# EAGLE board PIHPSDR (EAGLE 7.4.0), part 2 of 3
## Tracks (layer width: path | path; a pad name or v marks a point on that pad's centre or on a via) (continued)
N$321  (via drill 0.8 pad 1.93)
  other vias: 93.52,31.02
N$322  (via drill 0.8 pad 1.93)
  other vias: 93.52,28.48
N$323  (via drill 0.8 pad 1.93)
  other vias: 93.52,25.94
N$325  (via drill 0.8 pad 1.93)
  other vias: 96.06,119.92
N$326  (via drill 0.8 pad 1.93)
  other vias: 96.06,117.38
N$327  (via drill 0.8 pad 1.93)
  other vias: 96.06,114.84
N$328  (via drill 0.8 pad 1.93)
  other vias: 96.06,112.3
N$329  (via drill 0.8 pad 1.93)
  other vias: 96.06,109.76
N$330  (via drill 0.8 pad 1.93)
  other vias: 96.06,107.22
N$331  (via drill 0.8 pad 1.93)
  other vias: 96.06,104.68
N$332  (via drill 0.8 pad 1.93)
  other vias: 96.06,102.14
N$333  (via drill 0.8 pad 1.93)
  other vias: 96.06,99.6
N$334  (via drill 0.8 pad 1.93)
  other vias: 96.06,97.06
N$335  (via drill 0.8 pad 1.93)
  other vias: 96.06,94.52
N$336  (via drill 0.8 pad 1.93)
  other vias: 96.06,91.98
N$337  (via drill 0.8 pad 1.93)
  other vias: 96.06,89.44
N$338  (via drill 0.8 pad 1.93)
  other vias: 96.06,86.9
N$339  (via drill 0.8 pad 1.93)
  other vias: 96.06,84.36
N$340  (via drill 0.8 pad 1.93)
  other vias: 96.06,81.82
N$341  (via drill 0.8 pad 1.93)
  other vias: 96.06,79.28
N$342  (via drill 0.8 pad 1.93)
  other vias: 96.06,76.74
N$343  (via drill 0.8 pad 1.93)
  other vias: 96.06,74.2
N$344  (via drill 0.8 pad 1.93)
  other vias: 96.06,71.66
N$345  (via drill 0.8 pad 1.93)
  other vias: 96.06,69.12
N$346  (via drill 0.8 pad 1.93)
  other vias: 96.06,66.58
N$347  (via drill 0.8 pad 1.93)
  other vias: 96.06,64.04
N$348  (via drill 0.8 pad 1.93)
  other vias: 96.06,61.5
N$349  (via drill 0.8 pad 1.93)
  other vias: 96.06,58.96
N$350  (via drill 0.8 pad 1.93)
  other vias: 96.06,56.42
N$351  (via drill 0.8 pad 1.93)
  other vias: 96.06,53.88
N$352  (via drill 0.8 pad 1.93)
  other vias: 96.06,51.34
N$353  (via drill 0.8 pad 1.93)
  other vias: 96.06,48.8
N$354  (via drill 0.8 pad 1.93)
  other vias: 96.06,46.26
N$355  (via drill 0.8 pad 1.93)
  other vias: 96.06,43.72
N$356  (via drill 0.8 pad 1.93)
  other vias: 96.06,41.18
N$357  (via drill 0.8 pad 1.93)
  other vias: 96.06,38.64
N$358  (via drill 0.8 pad 1.93)
  other vias: 96.06,36.1
N$359  (via drill 0.8 pad 1.93)
  other vias: 96.06,33.56
N$360  (via drill 0.8 pad 1.93)
  other vias: 96.06,31.02
N$361  (via drill 0.8 pad 1.93)
  other vias: 96.06,28.48
N$362  (via drill 0.8 pad 1.93)
  other vias: 96.06,25.94
N$364  (via drill 0.8 pad 1.93)
  other vias: 98.6,119.92
N$365  (via drill 0.8 pad 1.93)
  other vias: 98.6,117.38
N$366  (via drill 0.8 pad 1.93)
  other vias: 98.6,114.84
N$367  (via drill 0.8 pad 1.93)
  other vias: 98.6,112.3
N$368  (via drill 0.8 pad 1.93)
  other vias: 98.6,109.76
N$369  (via drill 0.8 pad 1.93)
  other vias: 98.6,107.22
N$370  (via drill 0.8 pad 1.93)
  other vias: 98.6,104.68
N$371  (via drill 0.8 pad 1.93)
  other vias: 98.6,102.14
N$372  (via drill 0.8 pad 1.93)
  other vias: 98.6,99.6
N$373  (via drill 0.8 pad 1.93)
  other vias: 98.6,97.06
N$374  (via drill 0.8 pad 1.93)
  other vias: 98.6,94.52
N$375  (via drill 0.8 pad 1.93)
  other vias: 98.6,91.98
N$376  (via drill 0.8 pad 1.93)
  other vias: 98.6,89.44
N$377  (via drill 0.8 pad 1.93)
  other vias: 98.6,86.9
N$378  (via drill 0.8 pad 1.93)
  other vias: 98.6,84.36
N$379  (via drill 0.8 pad 1.93)
  other vias: 98.6,81.82
N$380  (via drill 0.8 pad 1.93)
  other vias: 98.6,79.28
N$381  (via drill 0.8 pad 1.93)
  other vias: 98.6,76.74
N$382  (via drill 0.8 pad 1.93)
  other vias: 98.6,74.2
N$383  (via drill 0.8 pad 1.93)
  other vias: 98.6,71.66
N$384  (via drill 0.8 pad 1.93)
  other vias: 98.6,69.12
N$385  (via drill 0.8 pad 1.93)
  other vias: 98.6,66.58
N$386  (via drill 0.8 pad 1.93)
  other vias: 98.6,64.04
N$387  (via drill 0.8 pad 1.93)
  other vias: 98.6,61.5
N$388  (via drill 0.8 pad 1.93)
  other vias: 98.6,58.96
N$389  (via drill 0.8 pad 1.93)
  other vias: 98.6,56.42
N$390  (via drill 0.8 pad 1.93)
  other vias: 98.6,53.88
N$391  (via drill 0.8 pad 1.93)
  other vias: 98.6,51.34
N$392  (via drill 0.8 pad 1.93)
  other vias: 98.6,48.8
N$393  (via drill 0.8 pad 1.93)
  other vias: 98.6,46.26
N$394  (via drill 0.8 pad 1.93)
  other vias: 98.6,43.72
N$395  (via drill 0.8 pad 1.93)
  other vias: 98.6,41.18
N$396  (via drill 0.8 pad 1.93)
  other vias: 98.6,38.64
N$397  (via drill 0.8 pad 1.93)
  other vias: 98.6,36.1
N$398  (via drill 0.8 pad 1.93)
  other vias: 98.6,33.56
N$399  (via drill 0.8 pad 1.93)
  other vias: 98.6,31.02
N$400  (via drill 0.8 pad 1.93)
  other vias: 98.6,28.48
N$401  (via drill 0.8 pad 1.93)
  other vias: 98.6,25.94
N$403  (via drill 0.8 pad 1.93)
  other vias: 103.68,119.92
N$404  (via drill 0.8 pad 1.93)
  other vias: 103.68,117.38
N$405  (via drill 0.8 pad 1.93)
  other vias: 103.68,114.84
N$406  (via drill 0.8 pad 1.93)
  other vias: 103.68,112.3
N$407  (via drill 0.8 pad 1.93)
  other vias: 103.68,109.76
N$408  (via drill 0.8 pad 1.93)
  other vias: 103.68,107.22
N$409  (via drill 0.8 pad 1.93)
  other vias: 103.68,104.68
N$410  (via drill 0.8 pad 1.93)
  other vias: 103.68,102.14
N$411  (via drill 0.8 pad 1.93)
  other vias: 103.68,99.6
N$412  (via drill 0.8 pad 1.93)
  other vias: 103.68,97.06
N$413  (via drill 0.8 pad 1.93)
  other vias: 103.68,94.52
N$414  (via drill 0.8 pad 1.93)
  other vias: 103.68,91.98
N$415  (via drill 0.8 pad 1.93)
  other vias: 103.68,89.44
N$416  (via drill 0.8 pad 1.93)
  other vias: 103.68,86.9
N$417  (via drill 0.8 pad 1.93)
  other vias: 103.68,84.36
N$418  (via drill 0.8 pad 1.93)
  other vias: 103.68,81.82
N$419  (via drill 0.8 pad 1.93)
  other vias: 103.68,79.28
N$420  (via drill 0.8 pad 1.93)
  other vias: 103.68,76.74
N$421  (via drill 0.8 pad 1.93)
  other vias: 103.68,74.2
N$422  (via drill 0.8 pad 1.93)
  other vias: 103.68,71.66
N$423  (via drill 0.8 pad 1.93)
  other vias: 103.68,69.12
N$424  (via drill 0.8 pad 1.93)
  other vias: 103.68,66.58
N$425  (via drill 0.8 pad 1.93)
  other vias: 103.68,64.04
N$426  (via drill 0.8 pad 1.93)
  other vias: 103.68,61.5
N$427  (via drill 0.8 pad 1.93)
  other vias: 103.68,58.96
N$428  (via drill 0.8 pad 1.93)
  other vias: 103.68,56.42
N$429  (via drill 0.8 pad 1.93)
  other vias: 103.68,53.88
N$430  (via drill 0.8 pad 1.93)
  other vias: 103.68,51.34
N$431  (via drill 0.8 pad 1.93)
  other vias: 103.68,48.8
N$432  (via drill 0.8 pad 1.93)
  other vias: 103.68,46.26
N$433  (via drill 0.8 pad 1.93)
  other vias: 103.68,43.72
N$434  (via drill 0.8 pad 1.93)
  other vias: 103.68,41.18
N$435  (via drill 0.8 pad 1.93)
  other vias: 103.68,38.64
N$436  (via drill 0.8 pad 1.93)
  other vias: 103.68,36.1
N$437  (via drill 0.8 pad 1.93)
  other vias: 103.68,33.56
N$438  (via drill 0.8 pad 1.93)
  other vias: 103.68,31.02
N$439  (via drill 0.8 pad 1.93)
  other vias: 103.68,28.48
N$440  (via drill 0.8 pad 1.93)
  other vias: 103.68,25.94
N$442  (via drill 0.8 pad 1.93)
  other vias: 101.14,119.92
N$443  (via drill 0.8 pad 1.93)
  other vias: 101.14,117.38
N$444  (via drill 0.8 pad 1.93)
  other vias: 101.14,114.84
N$445  (via drill 0.8 pad 1.93)
  other vias: 101.14,112.3
N$446  (via drill 0.8 pad 1.93)
  other vias: 101.14,109.76
N$447  (via drill 0.8 pad 1.93)
  other vias: 101.14,107.22
N$448  (via drill 0.8 pad 1.93)
  other vias: 101.14,104.68
N$449  (via drill 0.8 pad 1.93)
  other vias: 101.14,102.14
N$450  (via drill 0.8 pad 1.93)
  other vias: 101.14,99.6
N$451  (via drill 0.8 pad 1.93)
  other vias: 101.14,97.06
N$452  (via drill 0.8 pad 1.93)
  other vias: 101.14,94.52
N$453  (via drill 0.8 pad 1.93)
  other vias: 101.14,91.98
N$454  (via drill 0.8 pad 1.93)
  other vias: 101.14,89.44
N$455  (via drill 0.8 pad 1.93)
  other vias: 101.14,86.9
N$456  (via drill 0.8 pad 1.93)
  other vias: 101.14,84.36
N$457  (via drill 0.8 pad 1.93)
  other vias: 101.14,81.82
N$458  (via drill 0.8 pad 1.93)
  other vias: 101.14,79.28
N$459  (via drill 0.8 pad 1.93)
  other vias: 101.14,76.74
N$460  (via drill 0.8 pad 1.93)
  other vias: 101.14,74.2
N$461  (via drill 0.8 pad 1.93)
  other vias: 101.14,71.66
N$462  (via drill 0.8 pad 1.93)
  other vias: 101.14,69.12
N$463  (via drill 0.8 pad 1.93)
  other vias: 101.14,66.58
N$464  (via drill 0.8 pad 1.93)
  other vias: 101.14,64.04
N$465  (via drill 0.8 pad 1.93)
  other vias: 101.14,61.5
N$466  (via drill 0.8 pad 1.93)
  other vias: 101.14,58.96
N$467  (via drill 0.8 pad 1.93)
  other vias: 101.14,56.42
N$468  (via drill 0.8 pad 1.93)
  other vias: 101.14,53.88
N$469  (via drill 0.8 pad 1.93)
  other vias: 101.14,51.34
N$470  (via drill 0.8 pad 1.93)
  other vias: 101.14,48.8
N$471  (via drill 0.8 pad 1.93)
  other vias: 101.14,46.26
N$472  (via drill 0.8 pad 1.93)
  other vias: 101.14,43.72
N$473  (via drill 0.8 pad 1.93)
  other vias: 101.14,41.18
N$474  (via drill 0.8 pad 1.93)
  other vias: 101.14,38.64
N$475  (via drill 0.8 pad 1.93)
  other vias: 101.14,36.1
N$476  (via drill 0.8 pad 1.93)
  other vias: 101.14,33.56
N$477  (via drill 0.8 pad 1.93)
  other vias: 101.14,31.02
N$478  (via drill 0.8 pad 1.93)
  other vias: 101.14,28.48
N$479  (via drill 0.8 pad 1.93)
  other vias: 101.14,25.94
N$481  (via drill 0.8 pad 1.93)
  other vias: 106.22,119.92
N$482  (via drill 0.8 pad 1.93)
  other vias: 106.22,117.38
N$483  (via drill 0.8 pad 1.93)
  other vias: 106.22,114.84
N$484  (via drill 0.8 pad 1.93)
  other vias: 106.22,112.3
N$485  (via drill 0.8 pad 1.93)
  other vias: 106.22,109.76
N$486  (via drill 0.8 pad 1.93)
  other vias: 106.22,107.22
N$487  (via drill 0.8 pad 1.93)
  other vias: 106.22,104.68
N$488  (via drill 0.8 pad 1.93)
  other vias: 106.22,102.14
N$489  (via drill 0.8 pad 1.93)
  other vias: 106.22,99.6
N$490  (via drill 0.8 pad 1.93)
  other vias: 106.22,97.06
N$491  (via drill 0.8 pad 1.93)
  other vias: 106.22,94.52
N$492  (via drill 0.8 pad 1.93)
  other vias: 106.22,91.98
N$493  (via drill 0.8 pad 1.93)
  other vias: 106.22,89.44
N$494  (via drill 0.8 pad 1.93)
  other vias: 106.22,86.9
N$495  (via drill 0.8 pad 1.93)
  other vias: 106.22,84.36
N$496  (via drill 0.8 pad 1.93)
  other vias: 106.22,81.82
N$497  (via drill 0.8 pad 1.93)
  other vias: 106.22,79.28
N$498  (via drill 0.8 pad 1.93)
  other vias: 106.22,76.74
N$499  (via drill 0.8 pad 1.93)
  other vias: 106.22,74.2
N$500  (via drill 0.8 pad 1.93)
  other vias: 106.22,71.66
N$501  (via drill 0.8 pad 1.93)
  other vias: 106.22,69.12
N$502  (via drill 0.8 pad 1.93)
  other vias: 106.22,66.58
N$503  (via drill 0.8 pad 1.93)
  other vias: 106.22,64.04
N$504  (via drill 0.8 pad 1.93)
  other vias: 106.22,61.5
N$505  (via drill 0.8 pad 1.93)
  other vias: 106.22,58.96
N$506  (via drill 0.8 pad 1.93)
  other vias: 106.22,56.42
N$507  (via drill 0.8 pad 1.93)
  other vias: 106.22,53.88
N$508  (via drill 0.8 pad 1.93)
  other vias: 106.22,51.34
N$509  (via drill 0.8 pad 1.93)
  other vias: 106.22,48.8
N$510  (via drill 0.8 pad 1.93)
  other vias: 106.22,46.26
N$511  (via drill 0.8 pad 1.93)
  other vias: 106.22,43.72
N$512  (via drill 0.8 pad 1.93)
  other vias: 106.22,41.18
N$513  (via drill 0.8 pad 1.93)
  other vias: 106.22,38.64
N$514  (via drill 0.8 pad 1.93)
  other vias: 106.22,36.1
N$515  (via drill 0.8 pad 1.93)
  other vias: 106.22,33.56
N$516  (via drill 0.8 pad 1.93)
  other vias: 106.22,31.02
N$517  (via drill 0.8 pad 1.93)
  other vias: 106.22,28.48
N$518  (via drill 0.8 pad 1.93)
  other vias: 106.22,25.94
N$520  (via drill 0.8 pad 1.93)
  other vias: 108.76,119.92
N$521  (via drill 0.8 pad 1.93)
  other vias: 108.76,117.38
N$522  (via drill 0.8 pad 1.93)
  other vias: 108.76,114.84
N$523  (via drill 0.8 pad 1.93)
  other vias: 108.76,112.3
N$524  (via drill 0.8 pad 1.93)
  other vias: 108.76,109.76
N$525  (via drill 0.8 pad 1.93)
  other vias: 108.76,107.22
N$526  (via drill 0.8 pad 1.93)
  other vias: 108.76,104.68
N$527  (via drill 0.8 pad 1.93)
  other vias: 108.76,102.14
N$528  (via drill 0.8 pad 1.93)
  other vias: 108.76,99.6
N$529  (via drill 0.8 pad 1.93)
  other vias: 108.76,97.06
N$530  (via drill 0.8 pad 1.93)
  other vias: 108.76,94.52
N$531  (via drill 0.8 pad 1.93)
  other vias: 108.76,91.98
N$532  (via drill 0.8 pad 1.93)
  other vias: 108.76,89.44
N$533  (via drill 0.8 pad 1.93)
  other vias: 108.76,86.9
N$534  (via drill 0.8 pad 1.93)
  other vias: 108.76,84.36
N$535  (via drill 0.8 pad 1.93)
  other vias: 108.76,81.82
N$536  (via drill 0.8 pad 1.93)
  other vias: 108.76,79.28
N$537  (via drill 0.8 pad 1.93)
  other vias: 108.76,76.74
N$538  (via drill 0.8 pad 1.93)
  other vias: 108.76,74.2
N$539  (via drill 0.8 pad 1.93)
  other vias: 108.76,71.66
N$540  (via drill 0.8 pad 1.93)
  other vias: 108.76,69.12
N$541  (via drill 0.8 pad 1.93)
  other vias: 108.76,66.58
N$542  (via drill 0.8 pad 1.93)
  other vias: 108.76,64.04
N$543  (via drill 0.8 pad 1.93)
  other vias: 108.76,61.5
N$544  (via drill 0.8 pad 1.93)
  other vias: 108.76,58.96
N$545  (via drill 0.8 pad 1.93)
  other vias: 108.76,56.42
N$546  (via drill 0.8 pad 1.93)
  other vias: 108.76,53.88
N$547  (via drill 0.8 pad 1.93)
  other vias: 108.76,51.34
N$548  (via drill 0.8 pad 1.93)
  other vias: 108.76,48.8
N$549  (via drill 0.8 pad 1.93)
  other vias: 108.76,46.26
N$550  (via drill 0.8 pad 1.93)
  other vias: 108.76,43.72
N$551  (via drill 0.8 pad 1.93)
  other vias: 108.76,41.18
N$552  (via drill 0.8 pad 1.93)
  other vias: 108.76,38.64
N$553  (via drill 0.8 pad 1.93)
  other vias: 108.76,36.1
N$554  (via drill 0.8 pad 1.93)
  other vias: 108.76,33.56
N$555  (via drill 0.8 pad 1.93)
  other vias: 108.76,31.02
N$556  (via drill 0.8 pad 1.93)
  other vias: 108.76,28.48
N$557  (via drill 0.8 pad 1.93)
  other vias: 108.76,25.94
N$559  (via drill 0.8 pad 1.93)
  other vias: 111.3,119.92
N$560  (via drill 0.8 pad 1.93)
  other vias: 111.3,117.38
N$561  (via drill 0.8 pad 1.93)
  other vias: 111.3,114.84
N$562  (via drill 0.8 pad 1.93)
  other vias: 111.3,112.3
N$563  (via drill 0.8 pad 1.93)
  other vias: 111.3,109.76
N$564  (via drill 0.8 pad 1.93)
  other vias: 111.3,107.22
N$565  (via drill 0.8 pad 1.93)
  other vias: 111.3,104.68
N$566  (via drill 0.8 pad 1.93)
  other vias: 111.3,102.14
N$567  (via drill 0.8 pad 1.93)
  other vias: 111.3,99.6
N$568  (via drill 0.8 pad 1.93)
  other vias: 111.3,97.06
N$569  (via drill 0.8 pad 1.93)
  other vias: 111.3,94.52
N$570  (via drill 0.8 pad 1.93)
  other vias: 111.3,91.98
N$571  (via drill 0.8 pad 1.93)
  other vias: 111.3,89.44
N$572  (via drill 0.8 pad 1.93)
  other vias: 111.3,86.9
N$573  (via drill 0.8 pad 1.93)
  other vias: 111.3,84.36
N$574  (via drill 0.8 pad 1.93)
  other vias: 111.3,81.82
N$575  (via drill 0.8 pad 1.93)
  other vias: 111.3,79.28
N$576  (via drill 0.8 pad 1.93)
  other vias: 111.3,76.74
N$577  (via drill 0.8 pad 1.93)
  other vias: 111.3,74.2
N$578  (via drill 0.8 pad 1.93)
  other vias: 111.3,71.66
N$579  (via drill 0.8 pad 1.93)
  other vias: 111.3,69.12
N$580  (via drill 0.8 pad 1.93)
  other vias: 111.3,66.58
N$581  (via drill 0.8 pad 1.93)
  other vias: 111.3,64.04
N$582  (via drill 0.8 pad 1.93)
  other vias: 111.3,61.5
N$583  (via drill 0.8 pad 1.93)
  other vias: 111.3,58.96
N$584  (via drill 0.8 pad 1.93)
  other vias: 111.3,56.42
N$585  (via drill 0.8 pad 1.93)
  other vias: 111.3,53.88
N$586  (via drill 0.8 pad 1.93)
  other vias: 111.3,51.34
N$587  (via drill 0.8 pad 1.93)
  other vias: 111.3,48.8
N$588  (via drill 0.8 pad 1.93)
  other vias: 111.3,46.26
N$589  (via drill 0.8 pad 1.93)
  other vias: 111.3,43.72
N$590  (via drill 0.8 pad 1.93)
  other vias: 111.3,41.18
N$591  (via drill 0.8 pad 1.93)
  other vias: 111.3,38.64
N$592  (via drill 0.8 pad 1.93)
  other vias: 111.3,36.1
N$593  (via drill 0.8 pad 1.93)
  other vias: 111.3,33.56
N$594  (via drill 0.8 pad 1.93)
  other vias: 111.3,31.02
N$595  (via drill 0.8 pad 1.93)
  other vias: 111.3,28.48
N$596  (via drill 0.8 pad 1.93)
  other vias: 111.3,25.94
N$598  (via drill 0.8 pad 1.93)
  other vias: 113.84,119.92
N$599  (via drill 0.8 pad 1.93)
  other vias: 113.84,117.38
N$600  (via drill 0.8 pad 1.93)
  other vias: 113.84,114.84
N$601  (via drill 0.8 pad 1.93)
  other vias: 113.84,112.3
N$602  (via drill 0.8 pad 1.93)
  other vias: 113.84,109.76
N$603  (via drill 0.8 pad 1.93)
  other vias: 113.84,107.22
N$604  (via drill 0.8 pad 1.93)
  other vias: 113.84,104.68
N$605  (via drill 0.8 pad 1.93)
  other vias: 113.84,102.14
N$606  (via drill 0.8 pad 1.93)
  other vias: 113.84,99.6
N$607  (via drill 0.8 pad 1.93)
  other vias: 113.84,97.06
N$608  (via drill 0.8 pad 1.93)
  other vias: 113.84,94.52
N$609  (via drill 0.8 pad 1.93)
  other vias: 113.84,91.98
N$610  (via drill 0.8 pad 1.93)
  other vias: 113.84,89.44
N$611  (via drill 0.8 pad 1.93)
  other vias: 113.84,86.9
N$612  (via drill 0.8 pad 1.93)
  other vias: 113.84,84.36
N$613  (via drill 0.8 pad 1.93)
  other vias: 113.84,81.82
N$614  (via drill 0.8 pad 1.93)
  other vias: 113.84,79.28
N$615  (via drill 0.8 pad 1.93)
  other vias: 113.84,76.74
N$616  (via drill 0.8 pad 1.93)
  other vias: 113.84,74.2
N$617  (via drill 0.8 pad 1.93)
  other vias: 113.84,71.66
N$618  (via drill 0.8 pad 1.93)
  other vias: 113.84,69.12
N$619  (via drill 0.8 pad 1.93)
  other vias: 113.84,66.58
N$620  (via drill 0.8 pad 1.93)
  other vias: 113.84,64.04
N$621  (via drill 0.8 pad 1.93)
  other vias: 113.84,61.5
N$622  (via drill 0.8 pad 1.93)
  other vias: 113.84,58.96
N$623  (via drill 0.8 pad 1.93)
  other vias: 113.84,56.42
N$624  (via drill 0.8 pad 1.93)
  other vias: 113.84,53.88
N$625  (via drill 0.8 pad 1.93)
  other vias: 113.84,51.34
N$626  (via drill 0.8 pad 1.93)
  other vias: 113.84,48.8
N$627  (via drill 0.8 pad 1.93)
  other vias: 113.84,46.26
N$628  (via drill 0.8 pad 1.93)
  other vias: 113.84,43.72
N$629  (via drill 0.8 pad 1.93)
  other vias: 113.84,41.18
N$630  (via drill 0.8 pad 1.93)
  other vias: 113.84,38.64
N$631  (via drill 0.8 pad 1.93)
  other vias: 113.84,36.1
N$632  (via drill 0.8 pad 1.93)
  other vias: 113.84,33.56
N$633  (via drill 0.8 pad 1.93)
  other vias: 113.84,31.02
N$634  (via drill 0.8 pad 1.93)
  other vias: 113.84,28.48
N$635  (via drill 0.8 pad 1.93)
  other vias: 113.84,25.94
N$637  (via drill 0.8 pad 1.93)
  other vias: 116.38,119.92
N$638  (via drill 0.8 pad 1.93)
  other vias: 116.38,117.38
N$639  (via drill 0.8 pad 1.93)
  other vias: 116.38,114.84
N$640  (via drill 0.8 pad 1.93)
  other vias: 116.38,112.3
N$641  (via drill 0.8 pad 1.93)
  other vias: 116.38,109.76
N$642  (via drill 0.8 pad 1.93)
  other vias: 116.38,107.22
N$643  (via drill 0.8 pad 1.93)
  other vias: 116.38,104.68
N$644  (via drill 0.8 pad 1.93)
  other vias: 116.38,102.14
N$645  (via drill 0.8 pad 1.93)
  other vias: 116.38,99.6
N$646  (via drill 0.8 pad 1.93)
  other vias: 116.38,97.06
N$647  (via drill 0.8 pad 1.93)
  other vias: 116.38,94.52
N$648  (via drill 0.8 pad 1.93)
  other vias: 116.38,91.98
N$649  (via drill 0.8 pad 1.93)
  other vias: 116.38,89.44
N$650  (via drill 0.8 pad 1.93)
  other vias: 116.38,86.9
N$651  (via drill 0.8 pad 1.93)
  other vias: 116.38,84.36
N$652  (via drill 0.8 pad 1.93)
  other vias: 116.38,81.82
N$653  (via drill 0.8 pad 1.93)
  other vias: 116.38,79.28
N$654  (via drill 0.8 pad 1.93)
  other vias: 116.38,76.74
N$655  (via drill 0.8 pad 1.93)
  other vias: 116.38,74.2
N$656  (via drill 0.8 pad 1.93)
  other vias: 116.38,71.66
N$657  (via drill 0.8 pad 1.93)
  other vias: 116.38,69.12
N$658  (via drill 0.8 pad 1.93)
  other vias: 116.38,66.58
N$659  (via drill 0.8 pad 1.93)
  other vias: 116.38,64.04
N$660  (via drill 0.8 pad 1.93)
  other vias: 116.38,61.5
N$661  (via drill 0.8 pad 1.93)
  other vias: 116.38,58.96
N$662  (via drill 0.8 pad 1.93)
  other vias: 116.38,56.42
N$663  (via drill 0.8 pad 1.93)
  other vias: 116.38,53.88
N$664  (via drill 0.8 pad 1.93)
  other vias: 116.38,51.34
N$665  (via drill 0.8 pad 1.93)
  other vias: 116.38,48.8
N$666  (via drill 0.8 pad 1.93)
  other vias: 116.38,46.26
N$667  (via drill 0.8 pad 1.93)
  other vias: 116.38,43.72
N$668  (via drill 0.8 pad 1.93)
  other vias: 116.38,41.18
N$669  (via drill 0.8 pad 1.93)
  other vias: 116.38,38.64
N$670  (via drill 0.8 pad 1.93)
  other vias: 116.38,36.1
N$671  (via drill 0.8 pad 1.93)
  other vias: 116.38,33.56
N$672  (via drill 0.8 pad 1.93)
  other vias: 116.38,31.02
N$673  (via drill 0.8 pad 1.93)
  other vias: 116.38,28.48
N$674  (via drill 0.8 pad 1.93)
  other vias: 116.38,25.94
N$676  (via drill 0.8 pad 1.93)
  other vias: 118.92,119.92
N$677  (via drill 0.8 pad 1.93)
  other vias: 118.92,117.38
N$678  (via drill 0.8 pad 1.93)
  other vias: 118.92,114.84
N$679  (via drill 0.8 pad 1.93)
  other vias: 118.92,112.3
N$680  (via drill 0.8 pad 1.93)
  other vias: 118.92,109.76
N$681  (via drill 0.8 pad 1.93)
  other vias: 118.92,107.22
N$682  (via drill 0.8 pad 1.93)
  other vias: 118.92,104.68
N$683  (via drill 0.8 pad 1.93)
  other vias: 118.92,102.14
N$684  (via drill 0.8 pad 1.93)
  other vias: 118.92,99.6
N$685  (via drill 0.8 pad 1.93)
  other vias: 118.92,97.06
N$686  (via drill 0.8 pad 1.93)
  other vias: 118.92,94.52
N$687  (via drill 0.8 pad 1.93)
  other vias: 118.92,91.98
N$688  (via drill 0.8 pad 1.93)
  other vias: 118.92,89.44
N$689  (via drill 0.8 pad 1.93)
  other vias: 118.92,86.9
N$690  (via drill 0.8 pad 1.93)
  other vias: 118.92,84.36
N$691  (via drill 0.8 pad 1.93)
  other vias: 118.92,81.82
N$692  (via drill 0.8 pad 1.93)
  other vias: 118.92,79.28
N$693  (via drill 0.8 pad 1.93)
  other vias: 118.92,76.74
N$694  (via drill 0.8 pad 1.93)
  other vias: 118.92,74.2
N$695  (via drill 0.8 pad 1.93)
  other vias: 118.92,71.66
N$696  (via drill 0.8 pad 1.93)
  other vias: 118.92,69.12
N$697  (via drill 0.8 pad 1.93)
  other vias: 118.92,66.58
N$698  (via drill 0.8 pad 1.93)
  other vias: 118.92,64.04
N$699  (via drill 0.8 pad 1.93)
  other vias: 118.92,61.5
N$700  (via drill 0.8 pad 1.93)
  other vias: 118.92,58.96
N$701  (via drill 0.8 pad 1.93)
  other vias: 118.92,56.42
N$702  (via drill 0.8 pad 1.93)
  other vias: 118.92,53.88
N$703  (via drill 0.8 pad 1.93)
  other vias: 118.92,51.34
N$704  (via drill 0.8 pad 1.93)
  other vias: 118.92,48.8
N$705  (via drill 0.8 pad 1.93)
  other vias: 118.92,46.26
N$706  (via drill 0.8 pad 1.93)
  other vias: 118.92,43.72
N$707  (via drill 0.8 pad 1.93)
  other vias: 118.92,41.18
N$708  (via drill 0.8 pad 1.93)
  other vias: 118.92,38.64
N$709  (via drill 0.8 pad 1.93)
  other vias: 118.92,36.1
N$710  (via drill 0.8 pad 1.93)
  other vias: 118.92,33.56
N$711  (via drill 0.8 pad 1.93)
  other vias: 118.92,31.02
N$712  (via drill 0.8 pad 1.93)
  other vias: 118.92,28.48
N$713  (via drill 0.8 pad 1.93)
  other vias: 118.92,25.94
N$715  (via drill 0.8 pad 1.93)
  other vias: 121.46,119.92
N$716  (via drill 0.8 pad 1.93)
  other vias: 121.46,117.38
N$717  (via drill 0.8 pad 1.93)
  other vias: 121.46,114.84
N$718  (via drill 0.8 pad 1.93)
  other vias: 121.46,112.3
N$719  (via drill 0.8 pad 1.93)
  other vias: 121.46,109.76
N$720  (via drill 0.8 pad 1.93)
  other vias: 121.46,107.22
N$721  (via drill 0.8 pad 1.93)
  other vias: 121.46,104.68
N$722  (via drill 0.8 pad 1.93)
  other vias: 121.46,102.14
N$723  (via drill 0.8 pad 1.93)
  other vias: 121.46,99.6
N$724  (via drill 0.8 pad 1.93)
  other vias: 121.46,97.06
N$725  (via drill 0.8 pad 1.93)
  other vias: 121.46,94.52
N$726  (via drill 0.8 pad 1.93)
  other vias: 121.46,91.98
N$727  (via drill 0.8 pad 1.93)
  other vias: 121.46,89.44
N$728  (via drill 0.8 pad 1.93)
  other vias: 121.46,86.9
N$729  (via drill 0.8 pad 1.93)
  other vias: 121.46,84.36
N$730  (via drill 0.8 pad 1.93)
  other vias: 121.46,81.82
N$731  (via drill 0.8 pad 1.93)
  other vias: 121.46,79.28
N$732  (via drill 0.8 pad 1.93)
  other vias: 121.46,76.74
N$733  (via drill 0.8 pad 1.93)
  other vias: 121.46,74.2
N$734  (via drill 0.8 pad 1.93)
  other vias: 121.46,71.66
N$735  (via drill 0.8 pad 1.93)
  other vias: 121.46,69.12
N$736  (via drill 0.8 pad 1.93)
  other vias: 121.46,66.58
N$737  (via drill 0.8 pad 1.93)
  other vias: 121.46,64.04
N$738  (via drill 0.8 pad 1.93)
  other vias: 121.46,61.5
N$739  (via drill 0.8 pad 1.93)
  other vias: 121.46,58.96
N$740  (via drill 0.8 pad 1.93)
  other vias: 121.46,56.42
N$741  (via drill 0.8 pad 1.93)
  other vias: 121.46,53.88
N$742  (via drill 0.8 pad 1.93)
  other vias: 121.46,51.34
N$743  (via drill 0.8 pad 1.93)
  other vias: 121.46,48.8
N$744  (via drill 0.8 pad 1.93)
  other vias: 121.46,46.26
N$745  (via drill 0.8 pad 1.93)
  other vias: 121.46,43.72
N$746  (via drill 0.8 pad 1.93)
  other vias: 121.46,41.18
N$747  (via drill 0.8 pad 1.93)
  other vias: 121.46,38.64
N$748  (via drill 0.8 pad 1.93)
  other vias: 121.46,36.1
N$749  (via drill 0.8 pad 1.93)
  other vias: 121.46,33.56
N$750  (via drill 0.8 pad 1.93)
  other vias: 121.46,31.02
N$751  (via drill 0.8 pad 1.93)
  other vias: 121.46,28.48
N$752  (via drill 0.8 pad 1.93)
  other vias: 121.46,25.94
N$754  (via drill 0.8 pad 1.93)
  other vias: 126.54,119.92
N$755  (via drill 0.8 pad 1.93)
  other vias: 126.54,117.38
N$756  (via drill 0.8 pad 1.93)
  other vias: 126.54,114.84
N$757  (via drill 0.8 pad 1.93)
  other vias: 126.54,112.3
N$758  (via drill 0.8 pad 1.93)
  other vias: 126.54,109.76
N$759  (via drill 0.8 pad 1.93)
  other vias: 126.54,107.22
N$760  (via drill 0.8 pad 1.93)
  other vias: 126.54,104.68
N$761  (via drill 0.8 pad 1.93)
  other vias: 126.54,102.14
N$762  (via drill 0.8 pad 1.93)
  other vias: 126.54,99.6
N$763  (via drill 0.8 pad 1.93)
  other vias: 126.54,97.06
N$764  (via drill 0.8 pad 1.93)
  other vias: 126.54,94.52
N$765  (via drill 0.8 pad 1.93)
  other vias: 126.54,91.98
N$766  (via drill 0.8 pad 1.93)
  other vias: 126.54,89.44
N$767  (via drill 0.8 pad 1.93)
  other vias: 126.54,86.9
N$768  (via drill 0.8 pad 1.93)
  other vias: 126.54,84.36
N$769  (via drill 0.8 pad 1.93)
  other vias: 126.54,81.82
N$770  (via drill 0.8 pad 1.93)
  other vias: 126.54,79.28
N$771  (via drill 0.8 pad 1.93)
  other vias: 126.54,76.74
N$772  (via drill 0.8 pad 1.93)
  other vias: 126.54,74.2
N$773  (via drill 0.8 pad 1.93)
  other vias: 126.54,71.66
N$774  (via drill 0.8 pad 1.93)
  other vias: 126.54,69.12
N$775  (via drill 0.8 pad 1.93)
  other vias: 126.54,66.58
N$776  (via drill 0.8 pad 1.93)
  other vias: 126.54,64.04
N$777  (via drill 0.8 pad 1.93)
  other vias: 126.54,61.5
N$778  (via drill 0.8 pad 1.93)
  other vias: 126.54,58.96
N$779  (via drill 0.8 pad 1.93)
  other vias: 126.54,56.42
N$780  (via drill 0.8 pad 1.93)
  other vias: 126.54,53.88
N$781  (via drill 0.8 pad 1.93)
  other vias: 126.54,51.34
N$782  (via drill 0.8 pad 1.93)
  other vias: 126.54,48.8
N$783  (via drill 0.8 pad 1.93)
  other vias: 126.54,46.26
N$784  (via drill 0.8 pad 1.93)
  other vias: 126.54,43.72
N$785  (via drill 0.8 pad 1.93)
  other vias: 126.54,41.18
N$786  (via drill 0.8 pad 1.93)
  other vias: 126.54,38.64
N$787  (via drill 0.8 pad 1.93)
  other vias: 126.54,36.1
N$788  (via drill 0.8 pad 1.93)
  other vias: 126.54,33.56
N$789  (via drill 0.8 pad 1.93)
  other vias: 126.54,31.02
N$790  (via drill 0.8 pad 1.93)
  other vias: 126.54,28.48
N$791  (via drill 0.8 pad 1.93)
  other vias: 126.54,25.94
N$793  (via drill 0.8 pad 1.93)
  other vias: 124,119.92
N$794  (via drill 0.8 pad 1.93)
  other vias: 124,117.38
N$795  (via drill 0.8 pad 1.93)
  other vias: 124,114.84
N$796  (via drill 0.8 pad 1.93)
  other vias: 124,112.3
N$797  (via drill 0.8 pad 1.93)
  other vias: 124,109.76
N$798  (via drill 0.8 pad 1.93)
  other vias: 124,107.22
N$799  (via drill 0.8 pad 1.93)
  other vias: 124,104.68
N$800  (via drill 0.8 pad 1.93)
  other vias: 124,102.14
N$801  (via drill 0.8 pad 1.93)
  other vias: 124,99.6
N$802  (via drill 0.8 pad 1.93)
  other vias: 124,97.06
N$803  (via drill 0.8 pad 1.93)
  other vias: 124,94.52
N$804  (via drill 0.8 pad 1.93)
  other vias: 124,91.98
N$805  (via drill 0.8 pad 1.93)
  other vias: 124,89.44
N$806  (via drill 0.8 pad 1.93)
  other vias: 124,86.9
N$807  (via drill 0.8 pad 1.93)
  other vias: 124,84.36
N$808  (via drill 0.8 pad 1.93)
  other vias: 124,81.82
N$809  (via drill 0.8 pad 1.93)
  other vias: 124,79.28
N$810  (via drill 0.8 pad 1.93)
  other vias: 124,76.74
N$811  (via drill 0.8 pad 1.93)
  other vias: 124,74.2
N$812  (via drill 0.8 pad 1.93)
  other vias: 124,71.66
N$813  (via drill 0.8 pad 1.93)
  other vias: 124,69.12
N$814  (via drill 0.8 pad 1.93)
  other vias: 124,66.58
N$815  (via drill 0.8 pad 1.93)
  other vias: 124,64.04
N$816  (via drill 0.8 pad 1.93)
  other vias: 124,61.5
N$817  (via drill 0.8 pad 1.93)
  other vias: 124,58.96
N$818  (via drill 0.8 pad 1.93)
  other vias: 124,56.42
N$819  (via drill 0.8 pad 1.93)
  other vias: 124,53.88
N$820  (via drill 0.8 pad 1.93)
  other vias: 124,51.34
N$821  (via drill 0.8 pad 1.93)
  other vias: 124,48.8
N$822  (via drill 0.8 pad 1.93)
  other vias: 124,46.26
N$823  (via drill 0.8 pad 1.93)
  other vias: 124,43.72
N$824  (via drill 0.8 pad 1.93)
  other vias: 124,41.18
N$825  (via drill 0.8 pad 1.93)
  other vias: 124,38.64
N$826  (via drill 0.8 pad 1.93)
  other vias: 124,36.1
N$827  (via drill 0.8 pad 1.93)
  other vias: 124,33.56
N$828  (via drill 0.8 pad 1.93)
  other vias: 124,31.02
N$829  (via drill 0.8 pad 1.93)
  other vias: 124,28.48
N$830  (via drill 0.8 pad 1.93)
  other vias: 124,25.94
N$832  (via drill 0.8 pad 1.93)
  other vias: 129.08,119.92
N$833  (via drill 0.8 pad 1.93)
  other vias: 129.08,117.38
N$834  (via drill 0.8 pad 1.93)
  other vias: 129.08,114.84
N$835  (via drill 0.8 pad 1.93)
  other vias: 129.08,112.3
N$836  (via drill 0.8 pad 1.93)
  other vias: 129.08,109.76
N$837  (via drill 0.8 pad 1.93)
  other vias: 129.08,107.22
N$838  (via drill 0.8 pad 1.93)
  other vias: 129.08,104.68
N$839  (via drill 0.8 pad 1.93)
  other vias: 129.08,102.14
N$840  (via drill 0.8 pad 1.93)
  other vias: 129.08,99.6
N$841  (via drill 0.8 pad 1.93)
  other vias: 129.08,97.06
N$842  (via drill 0.8 pad 1.93)
  other vias: 129.08,94.52
N$843  (via drill 0.8 pad 1.93)
  other vias: 129.08,91.98
N$844  (via drill 0.8 pad 1.93)
  other vias: 129.08,89.44
N$845  (via drill 0.8 pad 1.93)
  other vias: 129.08,86.9
N$846  (via drill 0.8 pad 1.93)
  other vias: 129.08,84.36
N$847  (via drill 0.8 pad 1.93)
  other vias: 129.08,81.82
N$848  (via drill 0.8 pad 1.93)
  other vias: 129.08,79.28
N$849  (via drill 0.8 pad 1.93)
  other vias: 129.08,76.74
N$850  (via drill 0.8 pad 1.93)
  other vias: 129.08,74.2
N$851  (via drill 0.8 pad 1.93)
  other vias: 129.08,71.66
N$852  (via drill 0.8 pad 1.93)
  other vias: 129.08,69.12
N$853  (via drill 0.8 pad 1.93)
  other vias: 129.08,66.58
N$854  (via drill 0.8 pad 1.93)
  other vias: 129.08,64.04
N$855  (via drill 0.8 pad 1.93)
  other vias: 129.08,61.5
N$856  (via drill 0.8 pad 1.93)
  other vias: 129.08,58.96
N$857  (via drill 0.8 pad 1.93)
  other vias: 129.08,56.42
N$858  (via drill 0.8 pad 1.93)
  other vias: 129.08,53.88
N$859  (via drill 0.8 pad 1.93)
  other vias: 129.08,51.34
N$860  (via drill 0.8 pad 1.93)
  other vias: 129.08,48.8
N$861  (via drill 0.8 pad 1.93)
  other vias: 129.08,46.26
N$862  (via drill 0.8 pad 1.93)
  other vias: 129.08,43.72
N$863  (via drill 0.8 pad 1.93)
  other vias: 129.08,41.18
N$864  (via drill 0.8 pad 1.93)
  other vias: 129.08,38.64
N$865  (via drill 0.8 pad 1.93)
  other vias: 129.08,36.1
N$866  (via drill 0.8 pad 1.93)
  other vias: 129.08,33.56
N$867  (via drill 0.8 pad 1.93)
  other vias: 129.08,31.02
N$868  (via drill 0.8 pad 1.93)
  other vias: 129.08,28.48
N$869  (via drill 0.8 pad 1.93)
  other vias: 129.08,25.94
N$871  (via drill 0.8 pad 1.93)
  other vias: 131.62,119.92
N$872  (via drill 0.8 pad 1.93)
  other vias: 131.62,117.38
N$873  (via drill 0.8 pad 1.93)
  other vias: 131.62,114.84
N$874  (via drill 0.8 pad 1.93)
  other vias: 131.62,112.3
N$875  (via drill 0.8 pad 1.93)
  other vias: 131.62,109.76
N$876  (via drill 0.8 pad 1.93)
  other vias: 131.62,107.22
N$877  (via drill 0.8 pad 1.93)
  other vias: 131.62,104.68
N$878  (via drill 0.8 pad 1.93)
  other vias: 131.62,102.14
N$879  (via drill 0.8 pad 1.93)
  other vias: 131.62,99.6
N$880  (via drill 0.8 pad 1.93)
  other vias: 131.62,97.06
N$881  (via drill 0.8 pad 1.93)
  other vias: 131.62,94.52
N$882  (via drill 0.8 pad 1.93)
  other vias: 131.62,91.98
N$883  (via drill 0.8 pad 1.93)
  other vias: 131.62,89.44
N$884  (via drill 0.8 pad 1.93)
  other vias: 131.62,86.9
N$885  (via drill 0.8 pad 1.93)
  other vias: 131.62,84.36
N$886  (via drill 0.8 pad 1.93)
  other vias: 131.62,81.82
N$887  (via drill 0.8 pad 1.93)
  other vias: 131.62,79.28
N$888  (via drill 0.8 pad 1.93)
  other vias: 131.62,76.74
N$889  (via drill 0.8 pad 1.93)
  other vias: 131.62,74.2
N$890  (via drill 0.8 pad 1.93)
  other vias: 131.62,71.66
N$891  (via drill 0.8 pad 1.93)
  other vias: 131.62,69.12
N$892  (via drill 0.8 pad 1.93)
  other vias: 131.62,66.58
N$893  (via drill 0.8 pad 1.93)
  other vias: 131.62,64.04
N$894  (via drill 0.8 pad 1.93)
  other vias: 131.62,61.5
N$895  (via drill 0.8 pad 1.93)
  other vias: 131.62,58.96
N$896  (via drill 0.8 pad 1.93)
  other vias: 131.62,56.42
N$897  (via drill 0.8 pad 1.93)
  other vias: 131.62,53.88
N$898  (via drill 0.8 pad 1.93)
  other vias: 131.62,51.34
N$899  (via drill 0.8 pad 1.93)
  other vias: 131.62,48.8
N$900  (via drill 0.8 pad 1.93)
  other vias: 131.62,46.26
N$901  (via drill 0.8 pad 1.93)
  other vias: 131.62,43.72
N$902  (via drill 0.8 pad 1.93)
  other vias: 131.62,41.18
N$903  (via drill 0.8 pad 1.93)
  other vias: 131.62,38.64
N$904  (via drill 0.8 pad 1.93)
  other vias: 131.62,36.1
N$905  (via drill 0.8 pad 1.93)
  other vias: 131.62,33.56
N$906  (via drill 0.8 pad 1.93)
  other vias: 131.62,31.02
N$907  (via drill 0.8 pad 1.93)
  other vias: 131.62,28.48
N$908  (via drill 0.8 pad 1.93)
  other vias: 131.62,25.94
N$910  (via drill 0.8 pad 1.93)
  other vias: 134.16,119.92
N$911  (via drill 0.8 pad 1.93)
  other vias: 134.16,117.38
N$912  (via drill 0.8 pad 1.93)
  other vias: 134.16,114.84
N$913  (via drill 0.8 pad 1.93)
  other vias: 134.16,112.3
N$914  (via drill 0.8 pad 1.93)
  other vias: 134.16,109.76
N$915  (via drill 0.8 pad 1.93)
  other vias: 134.16,107.22
N$916  (via drill 0.8 pad 1.93)
  other vias: 134.16,104.68
N$917  (via drill 0.8 pad 1.93)
  other vias: 134.16,102.14
N$918  (via drill 0.8 pad 1.93)
  other vias: 134.16,99.6
N$919  (via drill 0.8 pad 1.93)
  other vias: 134.16,97.06
N$920  (via drill 0.8 pad 1.93)
  other vias: 134.16,94.52
N$921  (via drill 0.8 pad 1.93)
  other vias: 134.16,91.98
N$922  (via drill 0.8 pad 1.93)
  other vias: 134.16,89.44
N$923  (via drill 0.8 pad 1.93)
  other vias: 134.16,86.9
N$924  (via drill 0.8 pad 1.93)
  other vias: 134.16,84.36
N$925  (via drill 0.8 pad 1.93)
  other vias: 134.16,81.82
N$926  (via drill 0.8 pad 1.93)
  other vias: 134.16,79.28
N$927  (via drill 0.8 pad 1.93)
  other vias: 134.16,76.74
N$928  (via drill 0.8 pad 1.93)
  other vias: 134.16,74.2
N$929  (via drill 0.8 pad 1.93)
  other vias: 134.16,71.66
N$930  (via drill 0.8 pad 1.93)
  other vias: 134.16,69.12
N$931  (via drill 0.8 pad 1.93)
  other vias: 134.16,66.58
N$932  (via drill 0.8 pad 1.93)
  other vias: 134.16,64.04
N$933  (via drill 0.8 pad 1.93)
  other vias: 134.16,61.5
N$934  (via drill 0.8 pad 1.93)
  other vias: 134.16,58.96
N$935  (via drill 0.8 pad 1.93)
  other vias: 134.16,56.42
N$936  (via drill 0.8 pad 1.93)
  other vias: 134.16,53.88
N$937  (via drill 0.8 pad 1.93)
  other vias: 134.16,51.34
N$938  (via drill 0.8 pad 1.93)
  other vias: 134.16,48.8
N$939  (via drill 0.8 pad 1.93)
  other vias: 134.16,46.26
N$940  (via drill 0.8 pad 1.93)
  other vias: 134.16,43.72
N$941  (via drill 0.8 pad 1.93)
  other vias: 134.16,41.18
N$942  (via drill 0.8 pad 1.93)
  other vias: 134.16,38.64
N$943  (via drill 0.8 pad 1.93)
  other vias: 134.16,36.1
N$944  (via drill 0.8 pad 1.93)
  other vias: 134.16,33.56
N$945  (via drill 0.8 pad 1.93)
  other vias: 134.16,31.02
N$946  (via drill 0.8 pad 1.93)
  other vias: 134.16,28.48
N$947  (via drill 0.8 pad 1.93)
  other vias: 134.16,25.94
N$949  (via drill 0.8 pad 1.93)
  other vias: 136.7,119.92
N$950  (via drill 0.8 pad 1.93)
  other vias: 136.7,117.38
N$951  (via drill 0.8 pad 1.93)
  other vias: 136.7,114.84
N$952  (via drill 0.8 pad 1.93)
  other vias: 136.7,112.3
N$953  (via drill 0.8 pad 1.93)
  other vias: 136.7,109.76
N$954  (via drill 0.8 pad 1.93)
  other vias: 136.7,107.22
N$955  (via drill 0.8 pad 1.93)
  other vias: 136.7,104.68
N$956  (via drill 0.8 pad 1.93)
  other vias: 136.7,102.14
N$957  (via drill 0.8 pad 1.93)
  other vias: 136.7,99.6
N$958  (via drill 0.8 pad 1.93)
  other vias: 136.7,97.06
N$959  (via drill 0.8 pad 1.93)
  other vias: 136.7,94.52
N$960  (via drill 0.8 pad 1.93)
  other vias: 136.7,91.98
N$961  (via drill 0.8 pad 1.93)
  other vias: 136.7,89.44
N$962  (via drill 0.8 pad 1.93)
  other vias: 136.7,86.9
N$963  (via drill 0.8 pad 1.93)
  other vias: 136.7,84.36
N$964  (via drill 0.8 pad 1.93)
  other vias: 136.7,81.82
N$965  (via drill 0.8 pad 1.93)
  other vias: 136.7,79.28
N$966  (via drill 0.8 pad 1.93)
  other vias: 136.7,76.74
N$967  (via drill 0.8 pad 1.93)
  other vias: 136.7,74.2
N$968  (via drill 0.8 pad 1.93)
  other vias: 136.7,71.66
N$969  (via drill 0.8 pad 1.93)
  other vias: 136.7,69.12
N$970  (via drill 0.8 pad 1.93)
  other vias: 136.7,66.58
N$971  (via drill 0.8 pad 1.93)
  other vias: 136.7,64.04
N$972  (via drill 0.8 pad 1.93)
  other vias: 136.7,61.5
N$973  (via drill 0.8 pad 1.93)
  other vias: 136.7,58.96
N$974  (via drill 0.8 pad 1.93)
  other vias: 136.7,56.42
N$975  (via drill 0.8 pad 1.93)
  other vias: 136.7,53.88
N$976  (via drill 0.8 pad 1.93)
  other vias: 136.7,51.34
N$977  (via drill 0.8 pad 1.93)
  other vias: 136.7,48.8
N$978  (via drill 0.8 pad 1.93)
  other vias: 136.7,46.26
N$979  (via drill 0.8 pad 1.93)
  other vias: 136.7,43.72
N$980  (via drill 0.8 pad 1.93)
  other vias: 136.7,41.18
N$981  (via drill 0.8 pad 1.93)
  other vias: 136.7,38.64
N$982  (via drill 0.8 pad 1.93)
  other vias: 136.7,36.1
N$983  (via drill 0.8 pad 1.93)
  other vias: 136.7,33.56
N$984  (via drill 0.8 pad 1.93)
  other vias: 136.7,31.02
N$985  (via drill 0.8 pad 1.93)
  other vias: 136.7,28.48
N$986  (via drill 0.8 pad 1.93)
  other vias: 136.7,25.94
N$988  (via drill 0.8 pad 1.93)
  other vias: 139.24,119.92
N$989  (via drill 0.8 pad 1.93)
  other vias: 139.24,117.38
N$990  (via drill 0.8 pad 1.93)
  other vias: 139.24,114.84
N$991  (via drill 0.8 pad 1.93)
  other vias: 139.24,112.3
N$992  (via drill 0.8 pad 1.93)
  other vias: 139.24,109.76
N$993  (via drill 0.8 pad 1.93)
  other vias: 139.24,107.22
N$994  (via drill 0.8 pad 1.93)
  other vias: 139.24,104.68
N$995  (via drill 0.8 pad 1.93)
  other vias: 139.24,102.14
N$996  (via drill 0.8 pad 1.93)
  other vias: 139.24,99.6
N$997  (via drill 0.8 pad 1.93)
  other vias: 139.24,97.06
N$998  (via drill 0.8 pad 1.93)
  other vias: 139.24,94.52
N$999  (via drill 0.8 pad 1.93)
  other vias: 139.24,91.98
N$1000  (via drill 0.8 pad 1.93)
  other vias: 139.24,89.44
N$1001  (via drill 0.8 pad 1.93)
  other vias: 139.24,86.9
N$1002  (via drill 0.8 pad 1.93)
  other vias: 139.24,84.36
N$1003  (via drill 0.8 pad 1.93)
  other vias: 139.24,81.82
N$1004  (via drill 0.8 pad 1.93)
  other vias: 139.24,79.28
N$1005  (via drill 0.8 pad 1.93)
  other vias: 139.24,76.74
N$1006  (via drill 0.8 pad 1.93)
  other vias: 139.24,74.2
N$1007  (via drill 0.8 pad 1.93)
  other vias: 139.24,71.66
N$1008  (via drill 0.8 pad 1.93)
  other vias: 139.24,69.12
N$1009  (via drill 0.8 pad 1.93)
  other vias: 139.24,66.58
N$1010  (via drill 0.8 pad 1.93)
  other vias: 139.24,64.04
N$1011  (via drill 0.8 pad 1.93)
  other vias: 139.24,61.5
N$1012  (via drill 0.8 pad 1.93)
  other vias: 139.24,58.96
N$1013  (via drill 0.8 pad 1.93)
  other vias: 139.24,56.42
N$1014  (via drill 0.8 pad 1.93)
  other vias: 139.24,53.88
N$1015  (via drill 0.8 pad 1.93)
  other vias: 139.24,51.34
N$1016  (via drill 0.8 pad 1.93)
  other vias: 139.24,48.8
N$1017  (via drill 0.8 pad 1.93)
  other vias: 139.24,46.26
N$1018  (via drill 0.8 pad 1.93)
  other vias: 139.24,43.72
N$1019  (via drill 0.8 pad 1.93)
  other vias: 139.24,41.18
N$1020  (via drill 0.8 pad 1.93)
  other vias: 139.24,38.64
N$1021  (via drill 0.8 pad 1.93)
  other vias: 139.24,36.1
N$1022  (via drill 0.8 pad 1.93)
  other vias: 139.24,33.56
N$1023  (via drill 0.8 pad 1.93)
  other vias: 139.24,31.02
N$1024  (via drill 0.8 pad 1.93)
  other vias: 139.24,28.48
N$1025  (via drill 0.8 pad 1.93)
  other vias: 139.24,25.94
N$1027  (via drill 0.8 pad 1.93)
  other vias: 141.78,119.92
N$1028  (via drill 0.8 pad 1.93)
  other vias: 141.78,117.38
N$1029  (via drill 0.8 pad 1.93)
  other vias: 141.78,114.84
N$1030  (via drill 0.8 pad 1.93)
  other vias: 141.78,112.3
N$1031  (via drill 0.8 pad 1.93)
  other vias: 141.78,109.76
N$1032  (via drill 0.8 pad 1.93)
  other vias: 141.78,107.22
N$1033  (via drill 0.8 pad 1.93)
  other vias: 141.78,104.68
N$1034  (via drill 0.8 pad 1.93)
  other vias: 141.78,102.14
N$1035  (via drill 0.8 pad 1.93)
  other vias: 141.78,99.6
N$1036  (via drill 0.8 pad 1.93)
  other vias: 141.78,97.06
N$1037  (via drill 0.8 pad 1.93)
  other vias: 141.78,94.52
N$1038  (via drill 0.8 pad 1.93)
  other vias: 141.78,91.98
N$1039  (via drill 0.8 pad 1.93)
  other vias: 141.78,89.44
N$1040  (via drill 0.8 pad 1.93)
  other vias: 141.78,86.9
N$1041  (via drill 0.8 pad 1.93)
  other vias: 141.78,84.36
N$1042  (via drill 0.8 pad 1.93)
  other vias: 141.78,81.82
N$1043  (via drill 0.8 pad 1.93)
  other vias: 141.78,79.28
N$1044  (via drill 0.8 pad 1.93)
  other vias: 141.78,76.74
N$1045  (via drill 0.8 pad 1.93)
  other vias: 141.78,74.2
N$1046  (via drill 0.8 pad 1.93)
  other vias: 141.78,71.66
N$1047  (via drill 0.8 pad 1.93)
  other vias: 141.78,69.12
N$1048  (via drill 0.8 pad 1.93)
  other vias: 141.78,66.58
N$1049  (via drill 0.8 pad 1.93)
  other vias: 141.78,64.04
N$1050  (via drill 0.8 pad 1.93)
  other vias: 141.78,61.5
N$1051  (via drill 0.8 pad 1.93)
  other vias: 141.78,58.96
N$1052  (via drill 0.8 pad 1.93)
  other vias: 141.78,56.42
N$1053  (via drill 0.8 pad 1.93)
  other vias: 141.78,53.88
N$1054  (via drill 0.8 pad 1.93)
  other vias: 141.78,51.34
N$1055  (via drill 0.8 pad 1.93)
  other vias: 141.78,48.8
N$1056  (via drill 0.8 pad 1.93)
  other vias: 141.78,46.26
N$1057  (via drill 0.8 pad 1.93)
  other vias: 141.78,43.72
N$1058  (via drill 0.8 pad 1.93)
  other vias: 141.78,41.18
N$1059  (via drill 0.8 pad 1.93)
  other vias: 141.78,38.64
N$1060  (via drill 0.8 pad 1.93)
  other vias: 141.78,36.1
N$1061  (via drill 0.8 pad 1.93)
  other vias: 141.78,33.56
N$1062  (via drill 0.8 pad 1.93)
  other vias: 141.78,31.02
N$1063  (via drill 0.8 pad 1.93)
  other vias: 141.78,28.48
N$1064  (via drill 0.8 pad 1.93)
  other vias: 141.78,25.94
N$1066  (via drill 0.8 pad 1.93)
  other vias: 144.32,119.92
N$1067  (via drill 0.8 pad 1.93)
  other vias: 144.32,117.38
N$1068  (via drill 0.8 pad 1.93)
  other vias: 144.32,114.84
N$1069  (via drill 0.8 pad 1.93)
  other vias: 144.32,112.3
N$1070  (via drill 0.8 pad 1.93)
  other vias: 144.32,109.76
N$1071  (via drill 0.8 pad 1.93)
  other vias: 144.32,107.22
N$1072  (via drill 0.8 pad 1.93)
  other vias: 144.32,104.68
N$1073  (via drill 0.8 pad 1.93)
  other vias: 144.32,102.14
N$1074  (via drill 0.8 pad 1.93)
  other vias: 144.32,99.6
N$1075  (via drill 0.8 pad 1.93)
  other vias: 144.32,97.06
N$1076  (via drill 0.8 pad 1.93)
  other vias: 144.32,94.52
N$1077  (via drill 0.8 pad 1.93)
  other vias: 144.32,91.98
N$1078  (via drill 0.8 pad 1.93)
  other vias: 144.32,89.44
N$1079  (via drill 0.8 pad 1.93)
  other vias: 144.32,86.9
N$1080  (via drill 0.8 pad 1.93)
  other vias: 144.32,84.36
N$1081  (via drill 0.8 pad 1.93)
  other vias: 144.32,81.82
N$1082  (via drill 0.8 pad 1.93)
  other vias: 144.32,79.28
N$1083  (via drill 0.8 pad 1.93)
  other vias: 144.32,76.74
N$1084  (via drill 0.8 pad 1.93)
  other vias: 144.32,74.2
N$1085  (via drill 0.8 pad 1.93)
  other vias: 144.32,71.66
N$1086  (via drill 0.8 pad 1.93)
  other vias: 144.32,69.12
N$1087  (via drill 0.8 pad 1.93)
  other vias: 144.32,66.58
N$1088  (via drill 0.8 pad 1.93)
  other vias: 144.32,64.04
N$1089  (via drill 0.8 pad 1.93)
  other vias: 144.32,61.5
N$1090  (via drill 0.8 pad 1.93)
  other vias: 144.32,58.96
N$1091  (via drill 0.8 pad 1.93)
  other vias: 144.32,56.42
N$1092  (via drill 0.8 pad 1.93)
  other vias: 144.32,53.88
N$1093  (via drill 0.8 pad 1.93)
  other vias: 144.32,51.34
N$1094  (via drill 0.8 pad 1.93)
  other vias: 144.32,48.8
N$1095  (via drill 0.8 pad 1.93)
  other vias: 144.32,46.26
N$1096  (via drill 0.8 pad 1.93)
  other vias: 144.32,43.72
N$1097  (via drill 0.8 pad 1.93)
  other vias: 144.32,41.18
N$1098  (via drill 0.8 pad 1.93)
  other vias: 144.32,38.64
N$1099  (via drill 0.8 pad 1.93)
  other vias: 144.32,36.1
N$1100  (via drill 0.8 pad 1.93)
  other vias: 144.32,33.56
N$1101  (via drill 0.8 pad 1.93)
  other vias: 144.32,31.02
N$1102  (via drill 0.8 pad 1.93)
  other vias: 144.32,28.48
N$1103  (via drill 0.8 pad 1.93)
  other vias: 144.32,25.94
N$1105  (via drill 0.8 pad 1.93)
  other vias: 149.4,119.92
N$1106  (via drill 0.8 pad 1.93)
  other vias: 149.4,117.38
N$1107  (via drill 0.8 pad 1.93)
  other vias: 149.4,114.84
N$1108  (via drill 0.8 pad 1.93)
  other vias: 149.4,112.3
N$1109  (via drill 0.8 pad 1.93)
  other vias: 149.4,109.76
N$1110  (via drill 0.8 pad 1.93)
  other vias: 149.4,107.22
N$1111  (via drill 0.8 pad 1.93)
  other vias: 149.4,104.68
N$1112  (via drill 0.8 pad 1.93)
  other vias: 149.4,102.14
N$1113  (via drill 0.8 pad 1.93)
  other vias: 149.4,99.6
N$1114  (via drill 0.8 pad 1.93)
  other vias: 149.4,97.06
N$1115  (via drill 0.8 pad 1.93)
  other vias: 149.4,94.52
N$1116  (via drill 0.8 pad 1.93)
  other vias: 149.4,91.98
N$1117  (via drill 0.8 pad 1.93)
  other vias: 149.4,89.44
N$1118  (via drill 0.8 pad 1.93)
  other vias: 149.4,86.9
N$1119  (via drill 0.8 pad 1.93)
  other vias: 149.4,84.36
N$1120  (via drill 0.8 pad 1.93)
  other vias: 149.4,81.82
N$1121  (via drill 0.8 pad 1.93)
  other vias: 149.4,79.28
N$1122  (via drill 0.8 pad 1.93)
  other vias: 149.4,76.74
N$1123  (via drill 0.8 pad 1.93)
  other vias: 149.4,74.2
N$1124  (via drill 0.8 pad 1.93)
  other vias: 149.4,71.66
N$1125  (via drill 0.8 pad 1.93)
  other vias: 149.4,69.12
N$1126  (via drill 0.8 pad 1.93)
  other vias: 149.4,66.58
N$1127  (via drill 0.8 pad 1.93)
  other vias: 149.4,64.04
N$1128  (via drill 0.8 pad 1.93)
  other vias: 149.4,61.5
N$1129  (via drill 0.8 pad 1.93)
  other vias: 149.4,58.96
N$1130  (via drill 0.8 pad 1.93)
  other vias: 149.4,56.42
N$1131  (via drill 0.8 pad 1.93)
  other vias: 149.4,53.88
N$1132  (via drill 0.8 pad 1.93)
  other vias: 149.4,51.34
N$1133  (via drill 0.8 pad 1.93)
  other vias: 149.4,48.8
N$1134  (via drill 0.8 pad 1.93)
  other vias: 149.4,46.26
N$1135  (via drill 0.8 pad 1.93)
  other vias: 149.4,43.72
N$1136  (via drill 0.8 pad 1.93)
  other vias: 149.4,41.18
N$1137  (via drill 0.8 pad 1.93)
  other vias: 149.4,38.64
N$1138  (via drill 0.8 pad 1.93)
  other vias: 149.4,36.1
N$1139  (via drill 0.8 pad 1.93)
  other vias: 149.4,33.56
N$1140  (via drill 0.8 pad 1.93)
  other vias: 149.4,31.02
N$1141  (via drill 0.8 pad 1.93)
  other vias: 149.4,28.48
N$1142  (via drill 0.8 pad 1.93)
  other vias: 149.4,25.94
N$1144  (via drill 0.8 pad 1.93)
  other vias: 146.86,119.92
N$1145  (via drill 0.8 pad 1.93)
  other vias: 146.86,117.38
N$1146  (via drill 0.8 pad 1.93)
  other vias: 146.86,114.84
N$1147  (via drill 0.8 pad 1.93)
  other vias: 146.86,112.3
N$1148  (via drill 0.8 pad 1.93)
  other vias: 146.86,109.76
N$1149  (via drill 0.8 pad 1.93)
  other vias: 146.86,107.22
N$1150  (via drill 0.8 pad 1.93)
  other vias: 146.86,104.68
N$1151  (via drill 0.8 pad 1.93)
  other vias: 146.86,102.14
N$1152  (via drill 0.8 pad 1.93)
  other vias: 146.86,99.6
N$1153  (via drill 0.8 pad 1.93)
  other vias: 146.86,97.06
N$1154  (via drill 0.8 pad 1.93)
  other vias: 146.86,94.52
N$1155  (via drill 0.8 pad 1.93)
  other vias: 146.86,91.98
N$1156  (via drill 0.8 pad 1.93)
  other vias: 146.86,89.44
N$1157  (via drill 0.8 pad 1.93)
  other vias: 146.86,86.9
N$1158  (via drill 0.8 pad 1.93)
  other vias: 146.86,84.36
N$1159  (via drill 0.8 pad 1.93)
  other vias: 146.86,81.82
N$1160  (via drill 0.8 pad 1.93)
  other vias: 146.86,79.28
N$1161  (via drill 0.8 pad 1.93)
  other vias: 146.86,76.74
N$1162  (via drill 0.8 pad 1.93)
  other vias: 146.86,74.2
N$1163  (via drill 0.8 pad 1.93)
  other vias: 146.86,71.66
N$1164  (via drill 0.8 pad 1.93)
  other vias: 146.86,69.12
N$1165  (via drill 0.8 pad 1.93)
  other vias: 146.86,66.58
N$1166  (via drill 0.8 pad 1.93)
  other vias: 146.86,64.04
N$1167  (via drill 0.8 pad 1.93)
  other vias: 146.86,61.5
N$1168  (via drill 0.8 pad 1.93)
  other vias: 146.86,58.96
N$1169  (via drill 0.8 pad 1.93)
  other vias: 146.86,56.42
N$1170  (via drill 0.8 pad 1.93)
  other vias: 146.86,53.88
N$1171  (via drill 0.8 pad 1.93)
  other vias: 146.86,51.34
N$1172  (via drill 0.8 pad 1.93)
  other vias: 146.86,48.8
N$1173  (via drill 0.8 pad 1.93)
  other vias: 146.86,46.26
N$1174  (via drill 0.8 pad 1.93)
  other vias: 146.86,43.72
N$1175  (via drill 0.8 pad 1.93)
  other vias: 146.86,41.18
N$1176  (via drill 0.8 pad 1.93)
  other vias: 146.86,38.64
N$1177  (via drill 0.8 pad 1.93)
  other vias: 146.86,36.1
N$1178  (via drill 0.8 pad 1.93)
  other vias: 146.86,33.56
N$1179  (via drill 0.8 pad 1.93)
  other vias: 146.86,31.02
N$1180  (via drill 0.8 pad 1.93)
  other vias: 146.86,28.48
N$1181  (via drill 0.8 pad 1.93)
  other vias: 146.86,25.94
N$1183  (via drill 0.8 pad 1.93)
  other vias: 151.94,119.92
N$1184  (via drill 0.8 pad 1.93)
  other vias: 151.94,117.38
N$1185  (via drill 0.8 pad 1.93)
  other vias: 151.94,114.84
N$1186  (via drill 0.8 pad 1.93)
  other vias: 151.94,112.3
N$1187  (via drill 0.8 pad 1.93)
  other vias: 151.94,109.76
N$1188  (via drill 0.8 pad 1.93)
